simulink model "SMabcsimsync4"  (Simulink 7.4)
settings: Solver=ode45  StartTime=0.0  StopTime=10  MaxStep=2e-4  RelTol=1e-3
InitFcn:
  | smparamabcsync4
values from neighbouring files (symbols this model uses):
  Bm = 0.10    (= 0.1)    [IMabc2.m]    (also in imabcparam.m = 0.01; IMabcrun0.m = 0.01; IMabcrun1.m = 0.001; IMcur0.m = 1e-06)
  D = str2num(get(h,'string'))    [acttrcalc1.m]
  gam = 2*pi/3    (= 2.09439510239)    [IMabc2.m]    (also in IMabcf0.m; IMabcf1.m; imabcparam.m; IMabcrun0.m)
  H = 0.60    (= 0.6)    [IMabc2.m]    (also in IMcur0.m = 0.3; imdef0vec.m = 0.3; imdef1vec.m = 0.3; imdef2vec.m = 0.3)
  Lm = eval(get(hLm,'String'))    [im3d.m]    (also in IMabc2.m = 4.5; imabcparam.m = 0.0847; IMabcrun0.m = 0.0847; IMabcrun1.m = 0.0847)
  Lrr = [Lr   -Lm/2 -Lm/2    [IMabc2.m]    (also in IMabcf0.m = [Lr   -Lm1/2 -Lm1/2; IMabcf1.m = [Lr   -Lm1/2 -Lm1/2)
  Lss = [Ls   -Lm/2 -Lm/2    [IMabc2.m]    (also in IMabcf0.m = [Ls   -Lm1/2 -Lm1/2; IMabcf1.m = [Ls   -Lm1/2 -Lm1/2)
  R = str2num(get(h,'string'))    [acttrcalc1.m]    (also in IMabc2.m = diag([Rs Rs Rs Rr Rr Rr]); IMabcf0.m = diag([Rs Rs Rs Rr Rr Rr]); IMabcf1.m = diag([Rs Rs Rs Rr Rr Rr]); IMcurf0.m = diag([Rs Rs Rr Rr]))
  TLf = 1.27    [IMabc2.m]    (also in IMabcrun0.m = 2; IMabcrun1.m = 2; IMcur0.m = 0.8)
  Vs = abs(Vas)    [calc0.m]    (also in Ccurverun.m = 1; IMabc2.m = 1; IMabcrun0.m = Vll*sqrt(2/3); IMabcrun1.m = Vll*sqrt(2/3))
  wo = 2*pi*freq0    [calc0.m]    (also in IMabc2.m = 376.991118431; imabcparam.m = 376.991118431; IMabcrun0.m = 376.991118431; IMabcrun1.m = 376.991118431)
undefined symbols (not defined in the file or in its folder): ka, kf, Laf, Lakd, Lakq, Row, vector, vf

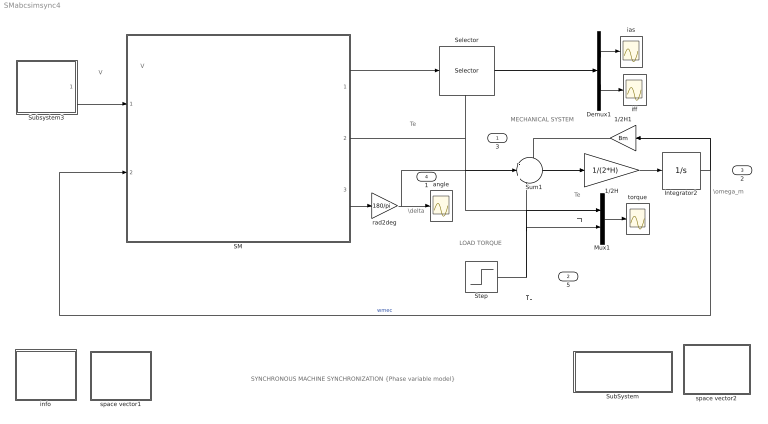
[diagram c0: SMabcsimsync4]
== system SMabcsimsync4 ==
  note: MECHANICAL SYSTEM
  note: Te
  note: Te
  note: TL
  note: LOAD TORQUE
  note: \omega_m
  note: V
  note: I
  note: \delta
  note: TL
  note: V
  note: SYNCHRONOUS MACHINE SYNCHRONIZATION {Phase variable model}
  1/2H : Gain  Gain=1/(2*H)  ParameterDataType=sfix(16)  ParameterScaling=2^0  OutDataType=sfix(16)  OutScaling=2^0
  1/2H1 : Gain  Gain=Bm  ParameterDataType=sfix(16)  ParameterScaling=2^0  OutDataType=sfix(16)  OutScaling=2^0
  Demux1 : Demux  Outputs=2
  Integrator2 : Integrator  InitialCondition=1
  Mux1 : Mux  Inputs=2
  SM : Subsystem
  Selector : Selector  InputPortWidth=6  IndexOptions=Index vector (dialog)  Indices=[1 4 ]  OutputSizes=1
  Step : Step  Time=4  After=TLf  SampleTime=0
  SubSystem : Subsystem
  Subsystem3 : Subsystem
  Sum1 : Sum  Inputs=-|+|-  OutDataType=sfix(16)  OutScaling=2^0
  angle : Scope
  ias : Scope
  iff : Scope
  info : Subsystem
  rad2deg : Gain  Gain=180/pi  ParameterDataType=sfix(16)  ParameterScaling=2^0  OutDataType=sfix(16)  OutScaling=2^0
  space vector1 : Subsystem
  space vector2 : Subsystem
  torque : Scope
  3 : Outport
  5 : Outport  Port=2
  2 : Outport  Port=3
  1 : Outport  Port=4
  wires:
  1/2H/1 -> Integrator2/1
  Integrator2/1 -> 1/2H1/1, SM/2(wm), 2/1  "wmec"
  Subsystem3/1(V) -> SM/1(V)
  Sum1/1 -> 1/2H/1
  Mux1/1 -> torque/1
  Demux1/2 -> iff/1
  Demux1/1 -> ias/1
  1/2H1/1 -> Sum1/1
  SM/1(I) -> Selector/1
  Selector/1 -> Demux1/1
  SM/2(Te) -> 3/1, Sum1/2, Mux1/1
  rad2deg/1 -> angle/1, 1/1
  SM/3(delta) -> rad2deg/1
  Step/1 -> 5/1, Mux1/2, Sum1/3

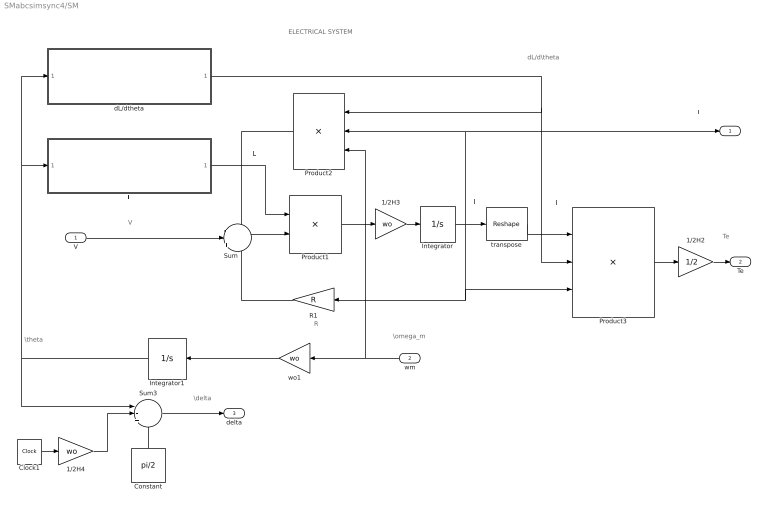
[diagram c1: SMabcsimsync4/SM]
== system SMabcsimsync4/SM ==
  note: \theta
  note: dL/d\theta
  note: L
  note: V
  note: ELECTRICAL SYSTEM
  note: I'
  note: I
  note: Te
  note: I
  note: \omega_m
  note: R
  note: \delta
  V : Inport  OutDataType=sfix(16)  OutScaling=2^0
  wm : Inport  Port=2  OutDataType=sfix(16)  OutScaling=2^0
  1/2H2 : Gain  Gain=1/2  ParameterDataType=sfix(16)  ParameterScaling=2^0  OutDataType=sfix(16)  OutScaling=2^0
  1/2H3 : Gain  Gain=wo  ParameterDataType=sfix(16)  ParameterScaling=2^0  OutDataType=sfix(16)  OutScaling=2^0
  1/2H4 : Gain  Gain=wo  ParameterDataType=sfix(16)  ParameterScaling=2^0  OutDataType=sfix(16)  OutScaling=2^0
  Clock1 : Clock
  Constant : Constant  Value=pi/2  OutDataType=sfix(16)  OutScaling=2^0
  Integrator : Integrator  InitialCondition=[0 ;0 ;0;kf* Vs/Lm;0 ;0 ]  ZeroCross=off
  Integrator1 : Integrator  InitialCondition=-ka*pi/2
  L : Subsystem
  Product1 : Product  Inputs=/*  Multiplication=Matrix(*)  OutDataType=sfix(16)  OutScaling=2^0
  Product2 : Product  Inputs=***  Multiplication=Matrix(*)  OutDataType=sfix(16)  OutScaling=2^0
  Product3 : Product  Inputs=3  Multiplication=Matrix(*)  OutDataType=sfix(16)  OutScaling=2^0
  R1 : Gain  Gain=R  Multiplication=Matrix(K*u)  ParameterDataType=sfix(16)  ParameterScaling=2^0  OutDataType=sfix(16)  OutScaling=2^0
  Sum : Sum  Inputs=-|+|-  OutDataType=sfix(16)  OutScaling=2^0
  Sum3 : Sum  Inputs=|-+-  OutDataType=sfix(16)  OutScaling=2^0
  dL/dtheta : Subsystem
  transpose : Reshape  OutputDimensionality=Row vector (2-D)  OutputDimensions=[1,6]
  wo1 : Gain  Gain=wo  ParameterDataType=sfix(16)  ParameterScaling=2^0  OutDataType=sfix(16)  OutScaling=2^0
  I : Outport
  Te : Outport  Port=2
  delta : Outport  Port=3
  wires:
  wo1/1 -> Integrator1/1
  R1/1 -> Sum/3
  1/2H3/1 -> Integrator/1
  Integrator/1 -> transpose/1, Product2/2, I/1, R1/1, Product3/3
  L/1(L) -> Product1/1
  Integrator1/1 -> dL/dtheta/1(theta1), L/1(theta), Sum3/1
  Product3/1 -> 1/2H2/1
  dL/dtheta/1(dLdtheta) -> Product2/1, Product3/2
  Product2/1 -> Sum/1
  transpose/1 -> Product3/1
  Sum/1 -> Product1/2
  Product1/1 -> 1/2H3/1
  wm/1 -> Product2/3, wo1/1
  V/1 -> Sum/2
  1/2H2/1 -> Te/1
  Clock1/1 -> 1/2H4/1
  1/2H4/1 -> Sum3/2
  Constant/1 -> Sum3/3
  Sum3/1 -> delta/1

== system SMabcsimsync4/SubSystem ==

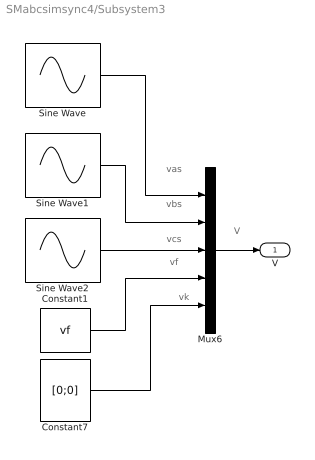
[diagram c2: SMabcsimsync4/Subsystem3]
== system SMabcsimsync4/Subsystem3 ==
  note: vk
  note: vf
  note: vcs
  note: vbs
  note: vas
  note: V
  Constant1 : Constant  Value=vf  VectorParams1D=off  OutDataType=sfix(16)  OutScaling=2^0
  Constant7 : Constant  Value=[0;0]  VectorParams1D=off  OutDataType=sfix(16)  OutScaling=2^0
  Mux6 : Mux  Inputs=5
  Sine Wave : Sin  Amplitude=Vs  Bias=0  Frequency=wo  Phase=pi/2  Samples=10  SampleTime=0
  Sine Wave1 : Sin  Amplitude=Vs  Bias=0  Frequency=wo  Phase=pi/2-gam  Samples=10  SampleTime=0
  Sine Wave2 : Sin  Amplitude=Vs  Bias=0  Frequency=wo  Phase=pi/2+gam  Samples=10  SampleTime=0
  V : Outport
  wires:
  Constant1/1 -> Mux6/4
  Constant7/1 -> Mux6/5
  Sine Wave/1 -> Mux6/1
  Sine Wave1/1 -> Mux6/2
  Sine Wave2/1 -> Mux6/3
  Mux6/1 -> V/1

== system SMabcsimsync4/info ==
  note: An alternator is running under open-circuit conditions when suddenly connected to a three-phase supply. Following synchronization, a step load is applied. The dynamic equations are expressed in matrix form in terms the phase variables, namely the stator currents ias, ibs, ics; the rotor field current iff; the d-axis and q-axis damper currents idk and iqk; the angular speed wm; and the displacement angle theta between stator as-axis and rotor direct axis. Torque, speed, and current responses are plotted as well as the torque angle. A Matlab script file for the identical system operation is given in the file >.
  note: SYNCHRONIZATION OF A SYNCHRONOUS GENERATOR (Phase variable model) [pu]

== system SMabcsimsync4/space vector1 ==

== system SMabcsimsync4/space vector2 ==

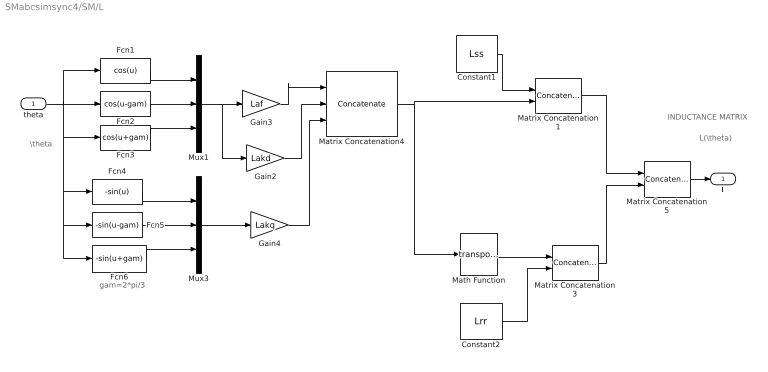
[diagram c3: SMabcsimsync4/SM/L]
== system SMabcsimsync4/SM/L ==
  note: INDUCTANCE MATRIX
  note: gam=2*pi/3
  note: \theta
  note: L(\theta)
  theta : Inport  OutDataType=sfix(16)  OutScaling=2^0
  Constant1 : Constant  Value=Lss  VectorParams1D=off  OutDataType=sfix(16)  OutScaling=2^0
  Constant2 : Constant  Value=Lrr  VectorParams1D=off  OutDataType=sfix(16)  OutScaling=2^0
  Fcn1 : Fcn  Expr=cos(u)
  Fcn2 : Fcn  Expr=cos(u-gam)
  Fcn3 : Fcn  Expr=cos(u+gam)
  Fcn4 : Fcn  Expr=-sin(u)
  Fcn5 : Fcn  Expr=-sin(u-gam)
  Fcn6 : Fcn  Expr=-sin(u+gam)
  Gain2 : Gain  Gain=Lakd  ParameterDataType=sfix(16)  ParameterScaling=2^0  OutDataType=sfix(16)  OutScaling=2^0
  Gain3 : Gain  Gain=Laf  ParameterDataType=sfix(16)  ParameterScaling=2^0  OutDataType=sfix(16)  OutScaling=2^0
  Gain4 : Gain  Gain=Lakq  ParameterDataType=sfix(16)  ParameterScaling=2^0  OutDataType=sfix(16)  OutScaling=2^0
  Math Function : Math  Operator=transpose
  Matrix Concatenation1 : Concatenate  Mode=Multidimensional array  ConcatenateDimension=2
  Matrix Concatenation3 : Concatenate  Mode=Multidimensional array  ConcatenateDimension=2
  Matrix Concatenation4 : Concatenate  NumInputs=3  Mode=Multidimensional array  ConcatenateDimension=2
  Matrix Concatenation5 : Concatenate  Mode=Multidimensional array
  Mux1 : Mux  Inputs=3
  Mux3 : Mux  Inputs=3
  L : Outport
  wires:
  Matrix Concatenation5/1 -> L/1
  Matrix Concatenation4/1 -> Matrix Concatenation1/2, Math Function/1
  Mux1/1 -> Gain3/1, Gain2/1
  Matrix Concatenation1/1 -> Matrix Concatenation5/1
  Constant1/1 -> Matrix Concatenation1/1
  Fcn3/1 -> Mux1/3
  Fcn2/1 -> Mux1/2
  Fcn1/1 -> Mux1/1
  theta/1 -> Fcn2/1, Fcn1/1, Fcn3/1, Fcn6/1, Fcn5/1, Fcn4/1
  Gain3/1 -> Matrix Concatenation4/1
  Gain2/1 -> Matrix Concatenation4/2
  Fcn5/1 -> Mux3/2
  Fcn4/1 -> Mux3/1
  Fcn6/1 -> Mux3/3
  Mux3/1 -> Gain4/1
  Gain4/1 -> Matrix Concatenation4/3
  Math Function/1 -> Matrix Concatenation3/1
  Constant2/1 -> Matrix Concatenation3/2
  Matrix Concatenation3/1 -> Matrix Concatenation5/2

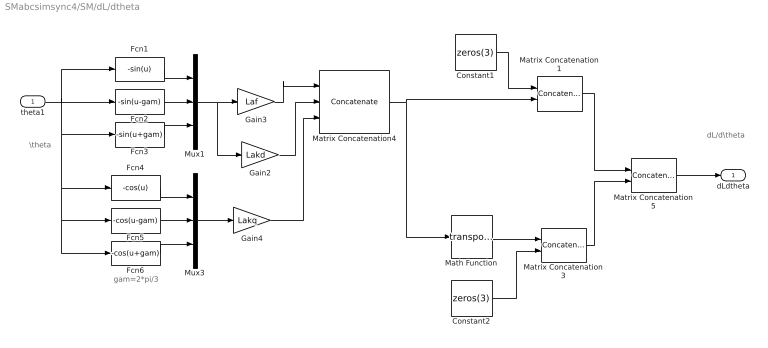
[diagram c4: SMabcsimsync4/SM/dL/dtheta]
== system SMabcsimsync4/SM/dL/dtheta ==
  note: dL/d\theta
  note: gam=2*pi/3
  note: \theta
  theta1 : Inport  OutDataType=sfix(16)  OutScaling=2^0
  Constant1 : Constant  Value=zeros(3)  VectorParams1D=off  OutDataType=sfix(16)  OutScaling=2^0
  Constant2 : Constant  Value=zeros(3)  VectorParams1D=off  OutDataType=sfix(16)  OutScaling=2^0
  Fcn1 : Fcn  Expr=-sin(u)
  Fcn2 : Fcn  Expr=-sin(u-gam)
  Fcn3 : Fcn  Expr=-sin(u+gam)
  Fcn4 : Fcn  Expr=-cos(u)
  Fcn5 : Fcn  Expr=-cos(u-gam)
  Fcn6 : Fcn  Expr=-cos(u+gam)
  Gain2 : Gain  Gain=Lakd  ParameterDataType=sfix(16)  ParameterScaling=2^0  OutDataType=sfix(16)  OutScaling=2^0
  Gain3 : Gain  Gain=Laf  ParameterDataType=sfix(16)  ParameterScaling=2^0  OutDataType=sfix(16)  OutScaling=2^0
  Gain4 : Gain  Gain=Lakq  ParameterDataType=sfix(16)  ParameterScaling=2^0  OutDataType=sfix(16)  OutScaling=2^0
  Math Function : Math  Operator=transpose
  Matrix Concatenation1 : Concatenate  Mode=Multidimensional array  ConcatenateDimension=2
  Matrix Concatenation3 : Concatenate  Mode=Multidimensional array  ConcatenateDimension=2
  Matrix Concatenation4 : Concatenate  NumInputs=3  Mode=Multidimensional array  ConcatenateDimension=2
  Matrix Concatenation5 : Concatenate  Mode=Multidimensional array
  Mux1 : Mux  Inputs=3
  Mux3 : Mux  Inputs=3
  dLdtheta : Outport
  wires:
  Matrix Concatenation5/1 -> dLdtheta/1
  Matrix Concatenation4/1 -> Matrix Concatenation1/2, Math Function/1
  Mux1/1 -> Gain3/1, Gain2/1
  Matrix Concatenation1/1 -> Matrix Concatenation5/1
  Constant1/1 -> Matrix Concatenation1/1
  Fcn3/1 -> Mux1/3
  Fcn2/1 -> Mux1/2
  Fcn1/1 -> Mux1/1
  theta1/1 -> Fcn2/1, Fcn1/1, Fcn3/1, Fcn6/1, Fcn5/1, Fcn4/1
  Gain3/1 -> Matrix Concatenation4/1
  Gain2/1 -> Matrix Concatenation4/2
  Fcn5/1 -> Mux3/2
  Fcn4/1 -> Mux3/1
  Fcn6/1 -> Mux3/3
  Mux3/1 -> Gain4/1
  Gain4/1 -> Matrix Concatenation4/3
  Math Function/1 -> Matrix Concatenation3/1
  Constant2/1 -> Matrix Concatenation3/2
  Matrix Concatenation3/1 -> Matrix Concatenation5/2
